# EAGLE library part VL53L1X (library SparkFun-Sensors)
STMicroelectronics VL53L1X - 400 cm IR Laser ToF Sensor VL53L1X is a state-of-the-art ToF laser-ranging sensor, enhancing the ST FlightSense product family. It is the fastest miniature ToF sensor currently on the market with accurate ranging up to 4 m and fast ranging frequency (up to 50 Hz). Housed in a miniature and reflowable package, it integrates a single photon avalanche diode (SPAD) receiving array, a 940 nm invisible laser Class 1 emitter, physical infrared filters, and optics to achieve the best ranging performance in various ambient lighting conditions with a range of cover window options.
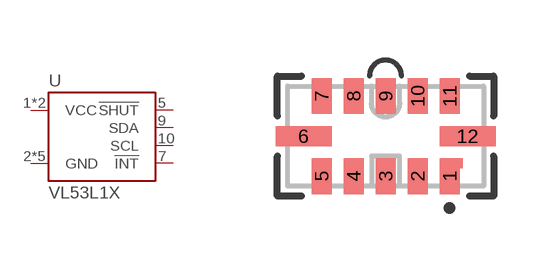
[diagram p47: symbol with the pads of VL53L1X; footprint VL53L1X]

Designator prefix U

## VL53L1XSMD (PROD_ID: IC-13960)  [VL53L1X]
1  VCC
2  GND
3  GND
4  GND
5  !SHUT
6  GND
7  !INT
9  SDA
10  SCL
11  VCC
12  GND

## Footprint VL53L1X (pad centres in mm)
LGA-12 - 12 pin LGA package for the V53L1x Specifications: Pin count: 12 Pin pitch: .8 mm Area: 4.8 mm x 2.4 mm Datasheet referenced for footprint
smd 0.5 x 0.9: 1 1.6,-1; 2 0.8,-1; 3 0,-1; 4 -0.8,-1; 5 -1.6,-1; 7 -1.6,1; 8 -0.8,1; 9 0,1; 10 0.8,1; 11 1.6,1
smd 1.4 x 0.5: 6 -2.05,0; 12 2.05,0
